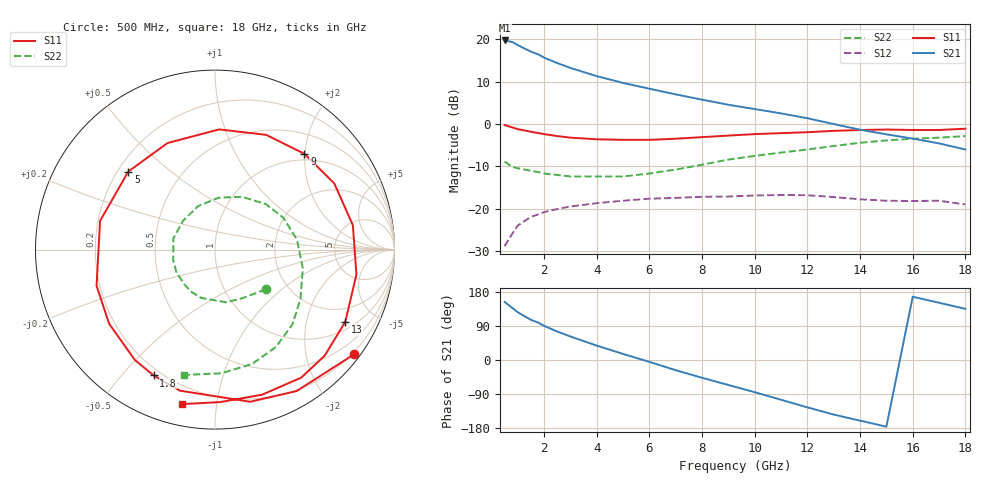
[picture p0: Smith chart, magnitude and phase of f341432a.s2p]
!ATF-34143
!S-PARAMETERS at Vds=2V  Id=20mA.  LAST UPDATED 01-29-99
# ghz s ma r 50
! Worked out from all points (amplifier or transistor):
!   23 points, 500 MHz to 18 GHz, reference 50 ohm
!   highest |S21| = 19.8 dB at 500 MHz (marker M1)
!   |S21| within 3 dB of that: start of sweep to 1.653 GHz
!   unconditionally stable (mu >= 1): 6.367 GHz to end of sweep
!   at 1.5 GHz: K = 0.34, MSG = 19.5 dB, |S12| = -21.9 dB
!   at 7 GHz: K = 1.05, MAG = 10.9 dB, |S12| = -17.5 dB
!   at 18 GHz: K = 1.51, MAG = 2.3 dB, |S12| = -19.0 dB
!   lowest NFmin = 0.10 dB at 500 MHz
!   S11 on the Smith chart (normalised r, x): 500 MHz: 0.15, -2.98; 1.8 GHz: 0.17, -0.61; 5 GHz: 0.24, +0.36; 9 GHz: 0.87, +1.99; 13 GHz: 1.31, -3.40; 18 GHz: 0.11, -0.80
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0.5  0.97 -37.0  9.718 153.0  0.036 68.0  0.36 -38.0
0.8  0.91 -60.0  9.29 137.0  0.051 56.0  0.31 -61.0
1  0.87 -77.0  8.545 126.0  0.063 48.0  0.3 -78.0
1.5  0.81 -104.0  7.181 106.0  0.08 34.0  0.28 -106.0
1.8  0.78 -116.0  6.603 98.0  0.086 28.0  0.27 -119.0
2  0.76 -126.0  6.088 90.0  0.091 23.0  0.26 -129.0
2.5  0.72 -145.0  5.253 75.0  0.099 14.0  0.25 -149.0
3  0.69 -163.0  4.602 62.0  0.106 6.0  0.24 -166.0
4  0.66 166.0  3.678 38.0  0.116 -8.0  0.24 165.0
5  0.65 138.0  3.058 16.0  0.124 -22.0  0.24 138.0
6  0.65 114.0  2.613 -5.0  0.131 -36.0  0.26 111.0
7  0.67 88.0  2.241 -27.0  0.134 -51.0  0.29 86.0
8  0.7 66.0  1.94 -47.0  0.138 -64.0  0.33 63.0
9  0.73 47.0  1.688 -66.0  0.139 -77.0  0.38 42.0
10  0.76 29.0  1.503 -85.0  0.143 -91.0  0.42 25.0
11  0.78 10.0  1.335 -105.0  0.145 -105.0  0.46 7.0
12  0.8 -10.0  1.17 -125.0  0.144 -121.0  0.5 -12.0
13  0.83 -29.0  0.999 -144.0  0.137 -135.0  0.55 -30.0
15  0.86 -56.0  0.755 -176.0  0.124 -158.0  0.64 -58.0
16  0.85 -72.0  0.672 167.0  0.123 -170.0  0.67 -72.0
17  0.85 -88.0  0.59 151.0  0.124 176.0  0.69 -87.0
18  0.88 -102.0  0.5 135.0  0.112 163.0  0.72 -104.0
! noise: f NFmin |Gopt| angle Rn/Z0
0.5  0.1  0.9  14  0.17
0.9  0.11  0.85  28  0.14
1.5  0.15  0.77  49  0.1
1.8  0.17  0.74  58  0.1
2.5  0.25  0.65  85  0.07
3  0.32  0.59  104  0.06
5  0.56  0.45  177  0.03
6  0.69  0.43  -148  0.05
8  0.95  0.47  -86  0.2
10  1.21  0.63  -42  0.5
